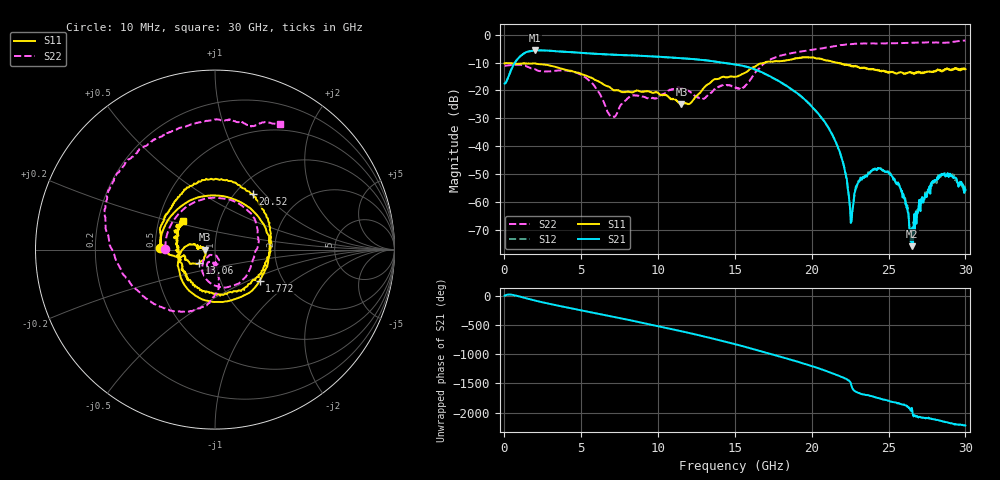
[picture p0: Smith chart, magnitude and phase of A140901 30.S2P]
!  2-Port S-parameters saved by WinCal
! VAR MeasName=S-Parameters (CALIBRATED_DATA) read from VNA (N5244A)
! VAR MeasDate=11/3/2014 9:29:16 AM
! VAR NAME=A140901 30
! VAR FILENAME=A140901 30.S2P
! VAR DATE=11/3/2014 9:29:16 AM
! VAR PHYS_PORTS=1,2
# Hz S RI R 50
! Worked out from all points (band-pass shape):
!   801 points, 10 MHz to 30 GHz, reference 50 ohm
!   highest |S21| = -5.58 dB at 1.959 GHz (marker M1); lowest = -75.8 dB at 26.51 GHz (marker M2)
!   |S21| within 3 dB of the highest: 879.7 MHz to 11.89 GHz (11.01 GHz wide, 172 % of centre)
!   lowest |S11| = -24.9 dB at 11.52 GHz (marker M3), VSWR 1.12, Z = 44.6 + j0.0457 ohm
!   |S11| at or under -10 dB: start of sweep to 16.94 GHz; 21.56051 GHz to 21.62783 GHz (67.33 MHz wide, 0.312 % of centre); 21.65 GHz to end of sweep
!   |S22| runs from -29.5 to -2.1 dB; largest |S21 - S12| = 0.0033
!   S11 on the Smith chart (normalised r, x): 10 MHz: 0.53, +0.01; 1.772 GHz: 1.53, -0.58; 13.06 GHz: 0.83, -0.13; 20.52 GHz: 1.20, +0.86; 30 GHz: 0.67, +0.23
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1e7  -0.3066 0.00812  0.133 0.00196  0.1336 0.00243  -0.2779 0.00595
7.5975e8  0.0637 0.2939  0.3397 0.00151  0.3395 0.00185  0.000287 0.2897
1.771912e9  0.2483 -0.1727  0.1789 -0.4797  0.1793 -0.4801  0.2417 0.0634
1.95935e9  0.1924 -0.2394  0.0746 -0.5207  0.0745 -0.5206  0.2413 0.0229
3.45885e9  -0.1734 -0.191  -0.4946 -0.0889  -0.4939 -0.0884  0.1758 -0.1434
5.033325e9  -0.195 -0.0233  -0.1307 0.4533  -0.1302 0.4529  -0.0263 -0.1865
7.170112e9  -0.0981 0.0233  0.4341 -0.0455  0.4334 -0.0451  0.00493 -0.0333
8.632125e9  -0.0993 0.00703  0.0395 -0.4202  0.0393 -0.4201  0.00155 -0.0813
1.001916e10  -0.0892 0.0119  -0.3833 -0.1262  -0.3826 -0.1254  0.00295 -0.0774
1.151866e10  -0.0567 0.00051  -0.1407 0.3517  -0.1404 0.3506  -0.0318 -0.1041
1.305565e10  -0.0895 -0.0761  0.3308 0.1107  0.3308 0.1094  -0.0124 -0.0722
1.5005e10  -0.1723 -0.0344  -0.0908 -0.2779  -0.092 -0.2767  -0.0366 -0.1076
1.691686e10  -0.3019 0.0821  -0.077 0.1867  -0.0758 0.1846  -0.0435 -0.3059
2.002832e10  0.0925 0.3815  -0.0302 -0.0405  -0.0297 -0.0408  -0.5236 -0.1127
2.051566e10  0.2114 0.3087  -0.035 -0.00675  -0.0349 -0.00756  -0.5581 -0.0393
2.182772e10  0.31 -0.0112  0.00359 0.00709  0.00359 0.00689  -0.6142 0.2023
2.257748e10  0.2118 -0.1686  -3.4e-05 -0.000444  -1.16e-05 -0.000434  -0.5831 0.3485
2.321476e10  0.07 -0.2414  -0.00132 0.00237  -0.00135 0.00231  -0.5086 0.4662
2.501416e10  -0.1672 -0.1236  0.00338 0.000141  0.00329 4.08e-05  -0.267 0.6501
2.651366e10  -0.201 -0.0316  -7.47e-05 -0.000143  -0.000192 -1.04e-05  -0.0678 0.7139
2.831306e10  -0.2263 0.0634  0.00256 0.00131  0.0027 0.00153  0.172 0.6982
3e10  -0.1793 0.1602  0.000869 -0.00141  0.00109 -0.00125  0.3612 0.6995
